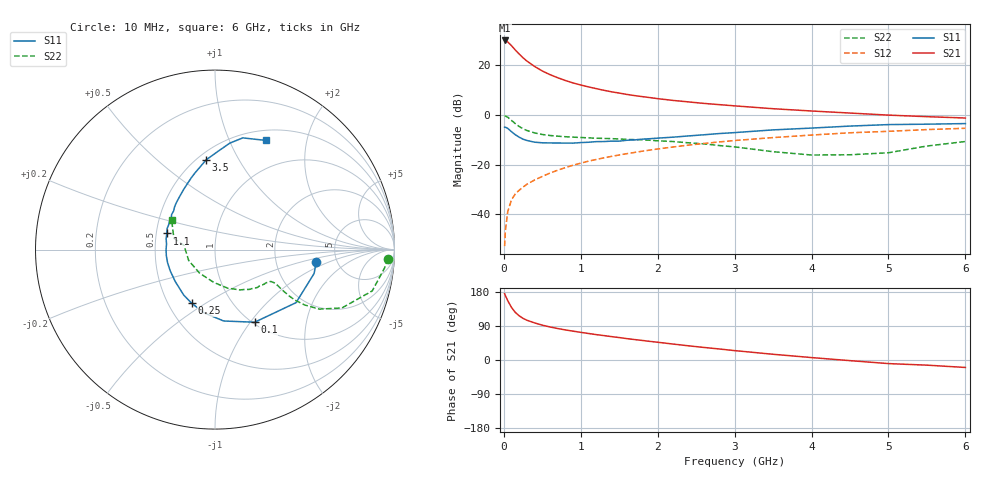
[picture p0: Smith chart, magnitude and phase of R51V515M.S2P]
! SIEMENS Small Signal Semiconductors
! BFR183
! Si NPN RF Bipolar Junction Transistor in SOT23
! VCE = 1.5 V  IC = 15 mA
! Common Emitter S-Parameters:  May  1996
# GHz  S  MA  R  50
!  f  S11  S21  S12  S22
! GHz  MAG  ANG  MAG  ANG  MAG  ANG  MAG  ANG
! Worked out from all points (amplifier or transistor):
!   36 points, 10 MHz to 6 GHz, reference 50 ohm
!   highest |S21| = 30.0 dB at 10 MHz (marker M1)
!   |S21| within 3 dB of that: start of sweep to 125.4 MHz
!   unconditionally stable (mu >= 1): 570.6 MHz to 2.485 GHz
!   at 250 MHz: K = 0.76, MSG = 26.0 dB, |S12| = -29.0 dB
!   at 1.4 GHz: K = 1.06, MAG = 11.5 dB, |S12| = -16.6 dB
!   at 6 GHz: K = 0.91, MSG = 2.1 dB, |S12| = -5.3 dB
!   S11 on the Smith chart (normalised r, x): 10 MHz: 3.47, -0.73; 100 MHz: 1.02, -1.05; 250 MHz: 0.65, -0.44; 1.1 GHz: 0.57, +0.11; 3.5 GHz: 0.55, +0.74; 6 GHz: 0.62, +1.38
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0.01  0.5686 -7.2  31.59 175.1  0.0023 85.9  0.9639 -3.0
0.02  0.5679 -13.6  31.27 170.1  0.0047 88.2  0.9501 -6.2
0.05  0.5397 -33.2  29.53 156.8  0.0113 77.5  0.906 -14.7
0.1  0.461 -61.4  24.83 138.6  0.0198 70.1  0.7783 -24.7
0.15  0.4006 -83.1  20.21 125.4  0.026 65.5  0.6693 -29.7
0.2  0.3577 -99.8  16.82 116.5  0.0307 64.8  0.5874 -31.7
0.25  0.3261 -113.4  14.13 109.8  0.0355 64.4  0.527 -32.3
0.3  0.3076 -124.5  12.16 104.9  0.0405 65.5  0.4875 -32.0
0.4  0.2839 -141.4  9.471 97.9  0.0493 66.2  0.4372 -31.0
0.5  0.2762 -154.7  7.682 91.9  0.0582 67.5  0.4054 -29.9
0.6  0.2742 -164.3  6.486 87.2  0.0679 68.0  0.3873 -29.3
0.7  0.2733 -172.6  5.622 83.1  0.0776 68.3  0.375 -29.3
0.8  0.2728 180.0  4.941 79.4  0.0875 67.9  0.3659 -29.5
0.9  0.2717 173.5  4.42 76.1  0.0979 67.8  0.3586 -29.7
1.1  0.2829 161.5  3.68 70.0  0.1179 67.2  0.3471 -31.6
1.3  0.2924 152.4  3.142 64.4  0.1376 65.7  0.3377 -33.6
1.6  0.3107 141.1  2.592 56.4  0.1672 63.1  0.3231 -38.2
2.2  0.3585 122.7  1.965 42.1  0.2275 56.9  0.2927 -49.3
3.5  0.502 95.7  1.338 15.1  0.3514 40.3  0.1827 -92.3
4.5  0.5988 82.1  1.095 -1.7  0.4392 27.3  0.1586 -157.5
5.5  0.6539 70.1  0.926 -13.6  0.509 15.4  0.2376 164.6
6  0.6722 64.8  0.87 -19.7  0.5409 7.7  0.293 145.6
